| TEXAS INSTRUMENTS INCORPORATED
| Standard Linear and Logic Group
| IBIS Model of SN74CB3Q3244
| 8 Bit Low Voltage High Band Width FET Bus Switch
| This file contains package information for the following:
|  TSSOP 20-pin (PW) package as [Component] CB3Q3244_PW
|  QFN 20-pin (RGY) package as [Component] CB3Q3244_RGY
|  TVSOP 20-pin (DGV) package as [Component] CB3Q3244_DGV
|  SSOP 20-pin (DBQ) package as [Component] CB3Q3244_DBQ
|  VFBGA 20-pin (GQN) package as [Component] CB3Q3244_GQN
| This device can be powered at the following Vccs:
|  3.3 volt Vcc
|  2.5 volt Vcc
| This file provides unique models under the [Model Selector] for each Vcc.
| For operation at a specific Vcc, select the appropriate model after each
| [Model Selector] keyword.
[IBIS Ver]   3.2
[Comment char]  |_char
[File Name]   sn74cb3q3244.ibs
[File Rev]   1.1 | b_die
[Date]   November 25, 2003
[Source]   Data created from TI-SPICE simulations at TI-SLL.
[Notes]   The following is an IBIS list for the CB3Q3244.
   Please contact sllibis@ti.com with questions and
   comments concerning SLL IBIS models.
   - Power-clamp data has been deleted since there is no
   power-clamp diode in the device.
   - The GQL package Component is commented out as
   there is different Series Pin Mapping.
[Disclaimer] Property of Texas Instruments Incorporated.  Unauthorized
   reproduction and/or distribution is strictly prohibited.
   This product is protected under copyright law.
   Created  2002, (C) Copyright  2002, Texas Instruments
   Incorporated, All Rights Reserved
   UNLESS THERE IS A SIGNED, WRITTEN AGREEMENT TO THE
   CONTRARY, TEXAS INSTRUMENTS (TI) IS PROVIDING THE IBIS
   MODELS  AND WITHOUT ANY WARRANTY, EXPRESSED OR
   IMPLIED.  TI assumes no liability for:
   1) the accuracy of the IBIS models provided to your
   company;
   2) the proper functioning of these IBIS Models in your
   design or for any resulting applications; or
   3) infringement of patents, copyrights or intellectual
   property rights resulting from your use of these IBIS
   models.
   TI provides IBIS Models as a service to our customers.
   You and your company shall not distribute, sell or give
   these models to anyone else without prior written
   permission from TI.
   TI reserves the right to make changes to our products or
   to discontinue any semiconductor product or service
   without notice, and advises our customers to obtain the
   latest version of relevant information to verify, before
   placing orders, that the information being relied on is
   current.
   Please be aware that your receipt and use of the IBIS
   information provided shall serve as acceptance of these
   terms and conditions.  If you do not accept these terms,
   you should return or destroy the IBIS models and any
   other accompanying information immediately.
| Component CB3Q3244_PW 20-pin TSSOP
[Component]   CB3Q3244_PW
[Manufacturer]   Texas Instruments, Inc.
[Package]
|   typ   min   max
R_pkg   5.000e-02   4.200e-02   6.000e-02
L_pkg   2.802e-09   2.248e-09   3.553e-09
C_pkg   3.170e-13   2.020e-13   4.430e-13
[Pin]   signal_name   model_name   R_pin   L_pin   C_pin
1   1NOE   CB3Q3244_IN   5.500e-02   3.461e-09   4.400e-13
2   1A1   CB3Q3244_IO   5.500e-02   3.150e-09   4.010e-13
3   2B4   CB3Q3244_IO   4.200e-02   2.619e-09   3.020e-13
4   1A2   CB3Q3244_IO   4.500e-02   2.273e-09   2.020e-13
5   2B3   CB3Q3244_IO   4.500e-02   2.248e-09   2.240e-13
6   1A3   CB3Q3244_IO   4.500e-02   2.273e-09   2.260e-13
7   2B2   CB3Q3244_IO   4.400e-02   2.323e-09   2.050e-13
8   1A4   CB3Q3244_IO   4.600e-02   2.704e-09   3.070e-13
9   2B1   CB3Q3244_IO   6.000e-02   3.265e-09   4.110e-13
10   GND   GND   5.700e-02   3.506e-09   4.360e-13
11   2A1   CB3Q3244_IO   5.800e-02   3.553e-09   4.370e-13
12   1B4   CB3Q3244_IO   5.800e-02   3.193e-09   4.050e-13
13   2A2   CB3Q3244_IO   4.200e-02   2.704e-09   3.110e-13
14   1B3   CB3Q3244_IO   4.600e-02   2.392e-09   2.100e-13
15   2A3   CB3Q3244_IO   4.700e-02   2.334e-09   2.290e-13
16   1B2   CB3Q3244_IO   4.700e-02   2.300e-09   2.270e-13
17   2A4   CB3Q3244_IO   4.700e-02   2.349e-09   2.070e-13
18   1B1   CB3Q3244_IO   4.500e-02   2.677e-09   3.060e-13
19   2NOE   CB3Q3244_IN   6.000e-02   3.235e-09   4.060e-13
20   VCC   POWER   5.600e-02   3.487e-09   4.430e-13
| Component CB3Q3244_RGY 20-pin QFN
[Component]   CB3Q3244_RGY
[Manufacturer]   Texas Instruments, Inc.
[Package]
|   typ   min   max
R_pkg   4.600e-02   3.500e-02   5.800e-02
L_pkg   1.131e-09   8.800e-10   1.396e-09
C_pkg   1.650e-13   1.420e-13   1.750e-13
[Pin]   signal_name   model_name   R_pin   L_pin   C_pin
1   1NOE   CB3Q3244_IN   5.300e-02   1.289e-09   1.420e-13
2   1A1   CB3Q3244_IO   5.800e-02   1.386e-09   1.720e-13
3   2B4   CB3Q3244_IO   4.600e-02   1.111e-09   1.730e-13
4   1A2   CB3Q3244_IO   3.900e-02   9.650e-10   1.610e-13
5   2B3   CB3Q3244_IO   3.500e-02   8.810e-10   1.650e-13
6   1A3   CB3Q3244_IO   3.500e-02   8.800e-10   1.650e-13
7   2B2   CB3Q3244_IO   3.900e-02   9.610e-10   1.610e-13
8   1A4   CB3Q3244_IO   4.500e-02   1.105e-09   1.720e-13
9   2B1   CB3Q3244_IO   5.800e-02   1.386e-09   1.720e-13
10   GND   GND   5.600e-02   1.352e-09   1.590e-13
11   2A1   CB3Q3244_IO   5.300e-02   1.287e-09   1.550e-13
12   1B4   CB3Q3244_IO   5.800e-02   1.396e-09   1.720e-13
13   2A2   CB3Q3244_IO   4.700e-02   1.129e-09   1.750e-13
14   1B3   CB3Q3244_IO   4.000e-02   9.760e-10   1.640e-13
15   2A3   CB3Q3244_IO   3.500e-02   8.840e-10   1.690e-13
16   1B2   CB3Q3244_IO   3.500e-02   8.810e-10   1.680e-13
17   2A4   CB3Q3244_IO   3.900e-02   9.670e-10   1.620e-13
18   1B1   CB3Q3244_IO   4.600e-02   1.118e-09   1.740e-13
19   2NOE   CB3Q3244_IN   5.800e-02   1.396e-09   1.750e-13
20   VCC   POWER   5.200e-02   1.276e-09   1.440e-13
| Component CB3Q3244_DGV 20-pin TVSOP
[Component]   CB3Q3244_DGV
[Manufacturer]   Texas Instruments, Inc.
[Package]
|   typ   min   max
R_pkg   4.400e-02   3.800e-02   4.800e-02
L_pkg   2.561e-09   2.236e-09   2.961e-09
C_pkg   3.420e-13   2.640e-13   4.460e-13
[Pin]   signal_name   model_name   R_pin   L_pin   C_pin
1   1NOE   CB3Q3244_IN   4.400e-02   2.935e-09   4.170e-13
2   1A1   CB3Q3244_IO   4.200e-02   2.869e-09   4.460e-13
3   2B4   CB3Q3244_IO   4.300e-02   2.399e-09   3.160e-13
4   1A2   CB3Q3244_IO   4.400e-02   2.236e-09   2.650e-13
5   2B3   CB3Q3244_IO   4.600e-02   2.278e-09   2.640e-13
6   1A3   CB3Q3244_IO   4.500e-02   2.274e-09   2.640e-13
7   2B2   CB3Q3244_IO   4.400e-02   2.285e-09   2.690e-13
8   1A4   CB3Q3244_IO   4.300e-02   2.452e-09   3.200e-13
9   2B1   CB3Q3244_IO   4.400e-02   2.900e-09   4.460e-13
10   GND   GND   4.400e-02   2.961e-09   4.180e-13
11   2A1   CB3Q3244_IO   4.500e-02   2.954e-09   4.180e-13
12   1B4   CB3Q3244_IO   4.200e-02   2.847e-09   4.430e-13
13   2A2   CB3Q3244_IO   4.500e-02   2.453e-09   3.190e-13
14   1B3   CB3Q3244_IO   4.500e-02   2.297e-09   2.690e-13
15   2A3   CB3Q3244_IO   4.800e-02   2.334e-09   2.680e-13
16   1B2   CB3Q3244_IO   4.800e-02   2.335e-09   2.670e-13
17   2A4   CB3Q3244_IO   4.600e-02   2.299e-09   2.680e-13
18   1B1   CB3Q3244_IO   4.600e-02   2.457e-09   3.200e-13
19   2NOE   CB3Q3244_IN   4.300e-02   2.848e-09   4.410e-13
20   VCC   POWER   3.800e-02   2.812e-09   4.080e-13
| Component CB3Q3244_DBQ 20-pin SSOP
[Component]   CB3Q3244_DBQ
[Manufacturer]   Texas Instruments, Inc.
[Package]
|   typ   min   max
R_pkg   3.900e-02   3.100e-02   5.000e-02
L_pkg   2.804e-09   2.292e-09   3.805e-09
C_pkg   2.940e-13   2.220e-13   4.170e-13
[Pin]   signal_name   model_name   R_pin   L_pin   C_pin
1   1NOE   CB3Q3244_IN   4.800e-02   3.760e-09   4.140e-13
2   1A1   CB3Q3244_IO   4.800e-02   3.053e-09   3.500e-13
3   2B4   CB3Q3244_IO   3.500e-02   2.506e-09   2.530e-13
4   1A2   CB3Q3244_IO   3.300e-02   2.368e-09   2.250e-13
5   2B3   CB3Q3244_IO   3.200e-02   2.302e-09   2.260e-13
6   1A3   CB3Q3244_IO   3.200e-02   2.303e-09   2.260e-13
7   2B2   CB3Q3244_IO   3.300e-02   2.368e-09   2.250e-13
8   1A4   CB3Q3244_IO   3.500e-02   2.506e-09   2.530e-13
9   2B1   CB3Q3244_IO   4.800e-02   3.053e-09   3.490e-13
10   GND   GND   4.200e-02   3.572e-09   4.040e-13
11   2A1   CB3Q3244_IO   4.700e-02   3.731e-09   4.140e-13
12   1B4   CB3Q3244_IO   4.900e-02   3.095e-09   3.550e-13
13   2A2   CB3Q3244_IO   4.000e-02   2.616e-09   2.590e-13
14   1B3   CB3Q3244_IO   3.300e-02   2.336e-09   2.220e-13
15   2A3   CB3Q3244_IO   3.300e-02   2.292e-09   2.250e-13
16   1B2   CB3Q3244_IO   3.300e-02   2.313e-09   2.270e-13
17   2A4   CB3Q3244_IO   3.100e-02   2.350e-09   2.230e-13
18   1B1   CB3Q3244_IO   4.000e-02   2.630e-09   2.600e-13
19   2NOE   CB3Q3244_IN   4.900e-02   3.109e-09   3.550e-13
20   VCC   POWER   5.000e-02   3.805e-09   4.170e-13
| Component CB3Q3244_GQN 20-pin VFBGA
|[Component]   CB3Q3244_GQN
|[Manufacturer]   Texas Instruments, Inc.
|[Package]
|   typ   min   max
|R_pkg   4.300e-02   3.300e-02   6.100e-02
|L_pkg   1.317e-09   0.896e-09   2.088e-09
|C_pkg   1.130e-13   0.640e-13   1.900e-13
|[Pin]   signal_name   model_name   R_pin   L_pin   C_pin
|A2   1NOE   CB3Q3244_IN   3.800e-02   1.199e-09   1.210e-13
|A1   1A1   CB3Q3244_IO   4.000e-02   1.067e-09   1.020e-13
|B3   2B4   CB3Q3244_IO   6.100e-02   1.999e-09   1.900e-13
|B1   1A2   CB3Q3244_IO   3.300e-02   0.963e-09   0.710e-13
|C2   2B3   CB3Q3244_IO   4.900e-02   1.523e-09   1.230e-13
|C1   1A3   CB3Q3244_IO   3.300e-02   0.896e-09   0.640e-13
|D3   2B2   CB3Q3244_IO   6.100e-02   1.899e-09   1.640e-13
|D1   1A4   CB3Q3244_IO   3.300e-02   0.898e-09   0.670e-13
|E2   2B1   CB3Q3244_IO   4.900e-02   1.514e-09   1.280e-13
|E1   GND   GND   3.600e-02   1.006e-09   0.940e-13
|E3   2A1   CB3Q3244_IO   4.900e-02   1.683e-09   1.460e-13
|E4   1B4   CB3Q3244_IO   3.300e-02   1.121e-09   0.890e-13
|D2   2A2   CB3Q3244_IO   6.100e-02   2.088e-09   1.730e-13
|D4   1B3   CB3Q3244_IO   3.300e-02   1.027e-09   0.710e-13
|C3   2A3   CB3Q3244_IO   4.900e-02   1.558e-09   1.240e-13
|C4   1B2   CB3Q3244_IO   3.300e-02   0.928e-09   0.670e-13
|B2   2A4   CB3Q3244_IO   6.100e-02   1.921e-09   1.770e-13
|B4   1B1   CB3Q3244_IO   3.300e-02   0.910e-09   0.770e-13
|A4   2NOE   CB3Q3244_IN   3.700e-02   0.990e-09   0.980e-13
|A3   VCC   POWER   3.500e-02   1.168e-09   1.190e-13
[Series Switch Groups]
| Function Group States
On  1 /   | 1A1-1A4->1B1-1B4 1NOE LOW
On  2 /   | 2A1-2A4->2B1-2B4 2NOE LOW
On  1 2 /   | Enable Both
[Series Pin Mapping]   pin_2   model_name   function_table_group
2   18   CB3Q3244_IO_33_S   1
| 2   18   CB3Q3244_IO_25_S   1
4   16   CB3Q3244_IO_33_S   1
| 4   16   CB3Q3244_IO_25_S   1
6   14   CB3Q3244_IO_33_S   1
| 6   14   CB3Q3244_IO_25_S   1
8   12   CB3Q3244_IO_33_S   1
| 8   12   CB3Q3244_IO_25_S   1
11   9   CB3Q3244_IO_33_S   2
| 11   9   CB3Q3244_IO_25_S   2
13   7   CB3Q3244_IO_33_S   2
| 13   7   CB3Q3244_IO_25_S   2
15   5   CB3Q3244_IO_33_S   2
| 15   5   CB3Q3244_IO_25_S   2
17   3   CB3Q3244_IO_33_S   2
| 17   3   CB3Q3244_IO_25_S   2
| Model CB3Q3244_IN
[Model Selector]   CB3Q3244_IN
CB3Q3244_IN_33   3.3 volt Vcc
CB3Q3244_IN_25   2.5 volt Vcc
| Model CB3Q3244_IO
[Model Selector]   CB3Q3244_IO
CB3Q3244_IO_33   3.3 volt Vcc
CB3Q3244_IO_25   2.5 volt Vcc
| Model CB3Q3244_IO_S
[Model Selector]   CB3Q3244_IO_S
CB3Q3244_IO_33_S   3.3 volt Vcc
CB3Q3244_IO_25_S   2.5 volt Vcc
[Model]   CB3Q3244_IO_33_S
Model_type  Series_switch
| variable   typ   min   max
C_comp   0   0   0
[Temperature Range]   40   100   -40
| Ambient temperature   25   85   -40
[Voltage range]   3.3   3   3.6
[On]
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[Off]
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[Model]   CB3Q3244_IO_25_S
Model_type  Series_switch
| variable   typ   min   max
C_comp   0   0   0
[Temperature Range]   40   100   -40
| Ambient temperature   25   85   -40
[Voltage range]   2.5   2.3   2.7
[On]
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[Off]
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| Models and submodels in the file (6): CB3Q3244_IN_33 (Input), CB3Q3244_IN_25 (Input), CB3Q3244_IO_33_S (Series_switch), CB3Q3244_IO_33 (Terminator), CB3Q3244_IO_25_S (Series_switch), CB3Q3244_IO_25 (Terminator)
